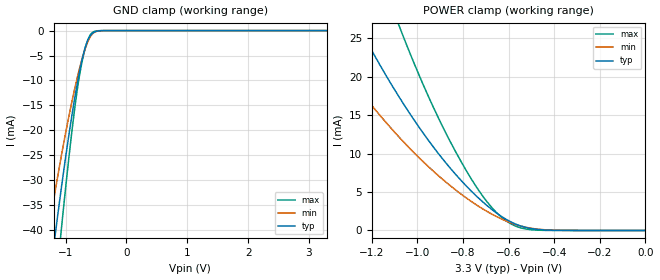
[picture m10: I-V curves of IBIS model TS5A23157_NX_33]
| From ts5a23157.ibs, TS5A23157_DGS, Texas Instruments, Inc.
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[Model]   TS5A23157_NX_33
Model_type  Terminator
| variable   typ   min   max
C_comp   5.76pF   5.18pF   6.22pF
| C_tri-state   5.76pF   5.18pF   6.22pF
[Temperature Range]   40   100   -40
| Ambient temperature   25   85   -40
[Voltage range]   3.3   3   3.6
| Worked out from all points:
|   GND clamp passes 1 mA (typ) near -0.59 V on its own axis
|   POWER clamp passes 1 mA (typ) near -0.58 V on its own axis
[GND Clamp]
| TS5A23157_NX_33
|   Voltage   I(typ)   I(min)   I(max)
-3.3V     -300.3mA   -237.2mA   -369.5mA
-1.3V     -53.63mA   -41.63mA   -69.16mA
-1.265V   -50.08mA   -38.97mA   -64.5mA
-1.16V    -39.81mA   -31.28mA   -50.88mA
-1.095V   -33.74mA   -26.75mA   -42.76mA
-1.065V   -31.03mA   -24.73mA   -39.11mA
-905mV    -17.6mA    -14.69mA   -20.97mA
-775mV    -8.424mA   -7.729mA   -9.183mA
-660mV    -2.697mA   -2.984mA   -2.725mA
-600mV    -1.13mA    -1.347mA   -953.5uA
-540mV    -369.6uA   -446.2uA   -224.8uA
3.3V      143.8pA    3.503uA    28.54pA
[POWER Clamp]
| TS5A23157_NX_33
|   Voltage   I(typ)   I(min)   I(max)
-3.3V     216.8mA    157.1mA    322.5mA
-1.45V    38.27mA    26.45mA    60.35mA
-1.265V   26.98mA    18.7mA     42.24mA
-1.24V    25.58mA    17.75mA    39.98mA
-1.07V    16.89mA    11.82mA    25.84mA
-950mV    11.66mA    8.256mA    17.32mA
-830mV    7.217mA    5.217mA    10.11mA
-730mV    4.161mA    3.114mA    5.161mA
-630mV    1.799mA    1.479mA    1.683mA
-570mV    837.1uA    780.8uA    568.1uA
-500mV    239.1uA    278.2uA    93.85uA
-48.03fV  143.8pA    899pA      34.56pA
